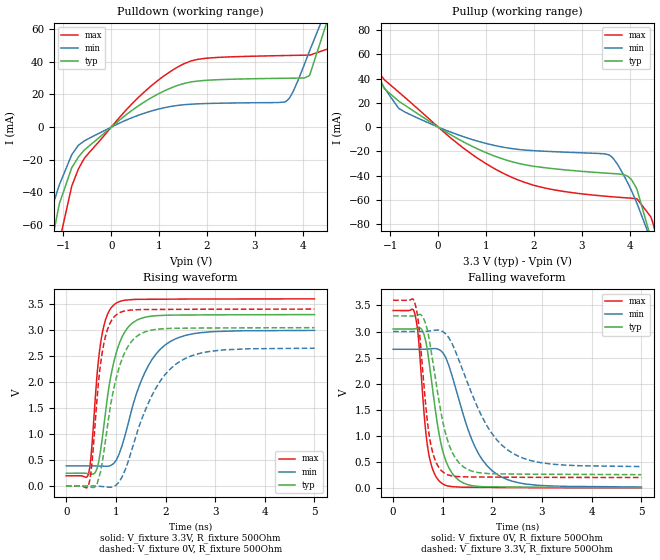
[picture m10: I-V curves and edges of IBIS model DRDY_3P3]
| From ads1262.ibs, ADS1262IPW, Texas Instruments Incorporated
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|   Model DRDY_3P3
[Model]   DRDY_3P3
Model_type   Output
Polarity   Non-Inverting
Enable   Active-Low
Vmeas = 1.65
Vref = 3.3
Cref = 15pF
Rref = 500
|   typ   min   max
|   (nom PVT)   (slow PVT)   (fast PVT)
C_comp   0.294p   0.276p   0.334p
|C_comp (ON state)   0.308p   0.292p   0.350p
|C_comp (OFF state)   0.294p   0.276p   0.334p
| Where   nom PVT is  Nominal Process, 3.3V, 27C
|   Fast PVT is Strong Process, 3.6V, -40C
|   Slow PVT is Weak Process, 3.0V, 125C
[Voltage Range]   3.3   3.0   3.6
[Temperature Range]   27   125   -40
[Pullup Reference]   3.3   3.0   3.6
[Pulldown Reference]   0   0   0
[Power Clamp Reference]   3.3   3.0   3.6
[GND Clamp Reference]   0   0   0
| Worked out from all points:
|   slope of the pulldown table from 0 to 0.495 V, typ, clamps not added: 42.9 ohm
|   slope of the pullup table from 0 to 0.495 V, typ, clamps not added: 42.9 ohm
|   falling waveform, V_fixture 0V, R_fixture 500Ohm: 20-80 % time 308ps typ, 599ps min, 189ps max; typ from 3.05 V to 0.005 V
|   rising waveform, V_fixture 3.3V, R_fixture 500Ohm: 20-80 % time 332ps typ, 592ps min, 197ps max; typ from 0.248 V to 3.3 V
|   rising waveform, V_fixture 0V, R_fixture 500Ohm: 20-80 % time 372ps typ, 706ps min, 215ps max; typ from 0 V to 3.05 V
|   falling waveform, V_fixture 3.3V, R_fixture 500Ohm: 20-80 % time 359ps typ, 772ps min, 212ps max; typ from 3.3 V to 0.254 V
[Pulldown]
|   Voltage   I(typ)   I(min)   I(max)
-3.3V     -480.7mA   -312.6mA   -682.1mA
-1.449V   -107.5mA   -71.63mA   -158.3mA
-1.201V   -64.41mA   -46.05mA   -93.85mA
-1.082V   -46.7mA    -35.15mA   -70mA
-825mV    -24.8mA    -16.87mA   -36.06mA
-547.8mV  -13.67mA   -8.239mA   -18.56mA
1.531V    26.78mA    13.71mA    38.94mA
3.64V     29.87mA    15.6mA     43.78mA
4.125V    31.31mA    45.54mA    44.04mA
4.561V    69.74mA    77.32mA    48.21mA
4.67V     80.48mA    84.46mA    59.99mA
6.59V     169.7mA    141.1mA    197.7mA
[Pullup]
|   Voltage   I(typ)   I(min)   I(max)
-3.3V     137.8mA    122.7mA    153.3mA
-2.132V   108.6mA    94.45mA    125.9mA
-1.726V   82.66mA    73.34mA    95.97mA
-1.122V   31.57mA    32.15mA    38.97mA
-825mV    21.4mA     15.43mA    28.92mA
541.2mV   -12.51mA   -8.128mA   -17.75mA
1.531V    -28.48mA   -17.72mA   -41.35mA
3.571V    -38.17mA   -23.09mA   -57.3mA
4.036V    -43.42mA   -52.51mA   -58.66mA
4.432V    -90.38mA   -92.27mA   -73.67mA
4.551V    -110.7mA   -105.7mA   -89.2mA
6.59V     -521.8mA   -378.6mA   -656.7mA
[Ramp]
R_load = 500
|   typ   min   max
dV/dt_r   1.82966/3.31793e-10   1.56307/5.91949e-10   2.04118/1.97288e-10
dV/dt_f   1.82618/3.0784e-10   1.58544/5.99265e-10   2.04155/1.89131e-10
[Falling Waveform]
V_fixture = 0V
V_fixture_min = 0V
V_fixture_max = 0V
R_fixture = 500Ohm
C_fixture = 0F
|   Time   V(typ)   V(min)   V(max)
0s        3.049V     2.66V      3.404V
437ps     3.052V     2.659V     3.34V
515.2ps   3.071V     2.659V     2.824V
595.3ps   3.006V     2.66V      1.781V
709.7ps   2.513V     2.666V     696.2mV
970.4ps   824.6mV    2.622V     94.47mV
1.331ns   140.4mV    1.675V     16.04mV
1.649ns   35.76mV    786.7mV    11.36mV
2.097ns   18.97mV    257.1mV    8.668mV
5ns       5.5mV      17.47mV    947.1uV
[Rising Waveform]
V_fixture = 3.3V
V_fixture_min = 3V
V_fixture_max = 3.6V
R_fixture = 500Ohm
C_fixture = 0F
|   Time   V(typ)   V(min)   V(max)
0s        247.9mV    388.3mV    197.7mV
454.5ps   237.8mV    389mV      259.7mV
595.3ps   280mV      387.1mV    1.826V
688.1ps   663.1mV    384.5mV    2.721V
794.9ps   1.443V     381.5mV    3.208V
970.4ps   2.43V      453.1mV    3.494V
1.189ns   2.981V     989.4mV    3.575V
1.575ns   3.243V     2.166V     3.591V
2.097ns   3.287V     2.781V     3.594V
5ns       3.297V     2.993V     3.6V
[Rising Waveform]
V_fixture = 0V
V_fixture_min = 0V
V_fixture_max = 0V
R_fixture = 500Ohm
C_fixture = 0F
|   Time   V(typ)   V(min)   V(max)
0s        1.422nV    3.318nV    1.147nV
454.5ps   -9.059mV   1.079mV    39.68mV
515.2ps   -24.37mV   1.223mV    416.2mV
623.1ps   45.73mV    -1.184mV   1.709V
731.3ps   494.5mV    -8.373mV   2.603V
1.035ns   2.176V     49.87mV    3.313V
1.417ns   2.877V     996.7mV    3.39V
1.797ns   3.011V     1.87V      3.396V
2.202ns   3.034V     2.34V      3.398V
5ns       3.046V     2.651V     3.403V
[Falling Waveform]
|Gnd
V_fixture = 3.3V
V_fixture_min = 3V
V_fixture_max = 3.6V
R_fixture = 500Ohm
C_fixture = 0F
|   Time   V(typ)   V(min)   V(max)
0s        3.3V       3V         3.6V
437ps     3.304V     3V         3.549V
515.2ps   3.326V     3V         3.144V
731.3ps   2.829V     3.011V     980.1mV
873.5ps   1.971V     3.028V     473mV
1.035ns   1.126V     2.974V     281.6mV
1.417ns   403.8mV    2.223V     213.1mV
1.897ns   275.8mV    1.179V     207.9mV
2.297ns   267.6mV    734.8mV    205.4mV
5ns       253.6mV    409.1mV    198.6mV
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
